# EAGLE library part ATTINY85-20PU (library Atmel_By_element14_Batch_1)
8-bit Microcontroller with In-System Programmable Flash
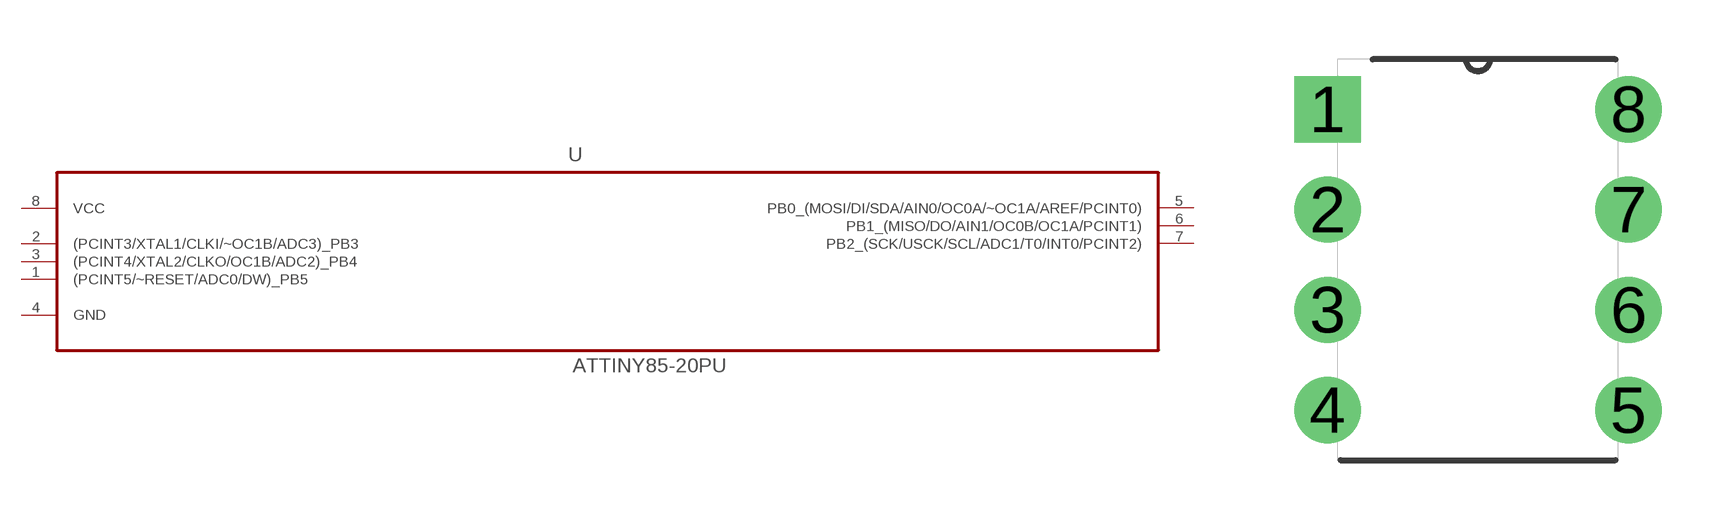
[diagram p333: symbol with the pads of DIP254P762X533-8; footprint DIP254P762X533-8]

Designator prefix U

## ATTINY85-20PU (MPN: ATTINY85-20PU; OC_FARNELL: 1455162; OC_NEWARK: 58M3796; PACKAGE: PDIP-8; SUPPLIER: Atmel)  [DIP254P762X533-8]
1  (PCINT5/~RESET/ADC0/DW)_PB5
2  (PCINT3/XTAL1/CLKI/~OC1B/ADC3)_PB3
3  (PCINT4/XTAL2/CLKO/OC1B/ADC2)_PB4
4  GND  pas
5  PB0_(MOSI/DI/SDA/AIN0/OC0A/~OC1A/AREF/PCINT0)
6  PB1_(MISO/DO/AIN1/OC0B/OC1A/PCINT1)
7  PB2_(SCK/USCK/SCL/ADC1/T0/INT0/PCINT2)
8  VCC  pwr

## Footprint DIP254P762X533-8 (pad centres in mm)
drill 1.118 square: 1 -7.62,7.62
drill 1.118: 2 -7.62,5.08; 3 -7.62,2.54; 4 -7.62,0; 5 0,0; 6 0,2.54; 7 0,5.08; 8 0,7.62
